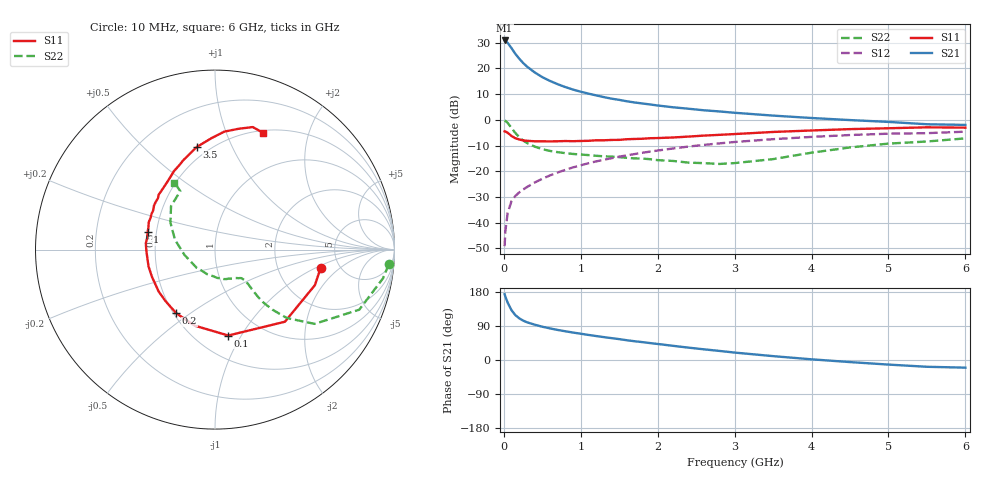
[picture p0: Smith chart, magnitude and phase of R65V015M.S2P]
! SIEMENS Small Signal Semiconductors
! BFR193
! Si NPN RF Bipolar Junction Transistor in SOT23
! VCE = 5 V  IC = 15 mA
! Common Emitter S-Parameters:  May  1996
# GHz  S  MA  R  50
!  f  S11  S21  S12  S22
! GHz  MAG  ANG  MAG  ANG  MAG  ANG  MAG  ANG
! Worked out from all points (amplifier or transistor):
!   36 points, 10 MHz to 6 GHz, reference 50 ohm
!   highest |S21| = 30.8 dB at 10 MHz (marker M1)
!   |S21| within 3 dB of that: start of sweep to 99.71 MHz
!   unconditionally stable (mu >= 1): 645.7 MHz to 1.889 GHz; 1.942 GHz to 2.036 GHz
!   at 250 MHz: K = 0.76, MSG = 24.6 dB, |S12| = -27.1 dB
!   at 1.4 GHz: K = 1.03, MAG = 10.5 dB, |S12| = -14.9 dB
!   at 6 GHz: K = 0.94, MSG = 1.3 dB, |S12| = -4.6 dB
!   S11 on the Smith chart (normalised r, x): 10 MHz: 3.58, -1.13; 100 MHz: 0.70, -0.88; 200 MHz: 0.52, -0.44; 1 GHz: 0.45, +0.10; 3.5 GHz: 0.43, +0.74; 6 GHz: 0.52, +1.36
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0.01  0.5976 -9.8  34.85 173.7  0.0035 87.4  0.9714 -4.9
0.02  0.5908 -19.6  34.39 167.3  0.0069 80.8  0.9497 -9.7
0.05  0.5597 -45.9  31.26 151.2  0.0156 72.9  0.8708 -22.6
0.1  0.4844 -81.2  24.64 131.3  0.0263 63.1  0.6924 -36.7
0.15  0.4385 -105.0  19.1 118.3  0.0332 59.9  0.5533 -43.6
0.2  0.4152 -121.3  15.43 110.1  0.0388 59.9  0.4624 -46.3
0.25  0.3977 -134.2  12.75 104.0  0.0441 60.7  0.3974 -47.6
0.3  0.3911 -143.4  10.86 99.6  0.0492 61.8  0.3548 -47.7
0.4  0.3826 -156.7  8.363 93.3  0.0604 63.7  0.302 -47.0
0.5  0.382 -165.9  6.751 87.8  0.0713 65.3  0.2687 -46.2
0.6  0.3801 -173.5  5.695 83.4  0.0831 66.1  0.2484 -45.9
0.7  0.3828 -179.9  4.921 79.3  0.0947 66.4  0.2351 -46.1
0.8  0.387 174.8  4.325 75.8  0.1065 66.2  0.2248 -46.7
1  0.388 165.5  3.515 69.3  0.1304 65.8  0.2116 -48.5
1.1  0.3906 161.9  3.227 66.2  0.1434 65.2  0.2061 -50.6
1.3  0.4001 154.0  2.761 60.4  0.1676 63.6  0.1952 -54.3
1.6  0.4194 144.1  2.289 52.1  0.204 60.7  0.1822 -62.6
2.2  0.4535 127.8  1.751 37.4  0.2772 53.6  0.1586 -85.1
3.5  0.5806 100.1  1.207 10.2  0.4201 34.7  0.1721 -169.8
4.5  0.6593 85.5  0.988 -5.5  0.5061 20.3  0.2903 148.8
5.5  0.7143 72.9  0.82 -17.9  0.5503 5.6  0.3788 120.7
6  0.7041 67.7  0.796 -20.2  0.5881 1.3  0.4357 121.2
